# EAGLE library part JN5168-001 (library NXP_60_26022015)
JenNet, ZigBee PRO and IEEE802.15.4 Module The JN5168-001-Myy family is a range of ultra low power, high performance surface mount modules targeted at IEEE 802.15.4, JenNet-IP, ZigBee Light Link, ZigBee Smart Energy and RF4CE networking applications, enabling users to realise products with minimum time to market and at the lowest cost. They remove the need for expensive and lengthy development of custom RF board designs and test suites. The modules use NXP’s JN5168 wireless microcontroller to provide a comprehensive solution with large memory, high CPU and radio performance and all RF components included. All that is required to develop and manufacture wireless control or sensing products is to connect a power supply and peripherals such as switches, actuators and sensors, considerably simplifying product development. Four module variants are available: JN5168-001-M00 with an integrated antenna, JN5168-001- M03 with an antenna connector and the JN5168-001-M05 and M06 with an antenna connector, power amplifier and LNA for extended range. The JN5168-001-M05 output power has been optimised for use in Europe and Asia. AAL Eindhoven MK
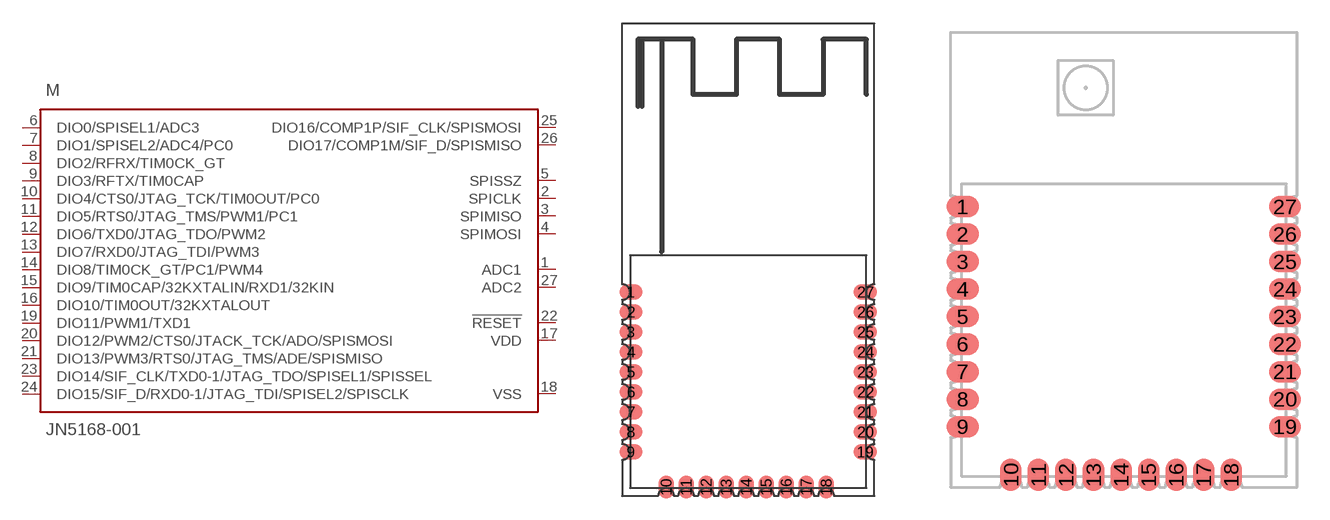
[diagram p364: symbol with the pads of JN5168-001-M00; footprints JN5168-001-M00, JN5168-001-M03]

Designator prefix M

## JN5168-001-M00 (DIO2: OK; DIO3: OK)  [JN5168-001-M00]
1  ADC1  pas
2  SPICLK  out
3  SPIMISO  in
4  SPIMOSI  in
5  SPISSZ  out
6  DIO0/SPISEL1/ADC3
7  DIO1/SPISEL2/ADC4/PC0
8  DIO2/RFRX/TIM0CK_GT
9  DIO3/RFTX/TIM0CAP
10  DIO4/CTS0/JTAG_TCK/TIM0OUT/PC0
11  DIO5/RTS0/JTAG_TMS/PWM1/PC1
12  DIO6/TXD0/JTAG_TDO/PWM2
13  DIO7/RXD0/JTAG_TDI/PWM3
14  DIO8/TIM0CK_GT/PC1/PWM4
15  DIO9/TIM0CAP/32KXTALIN/RXD1/32KIN
16  DIO10/TIM0OUT/32KXTALOUT
17  VDD
18  VSS  pwr
19  DIO11/PWM1/TXD1
20  DIO12/PWM2/CTS0/JTACK_TCK/ADO/SPISMOSI
21  DIO13/PWM3/RTS0/JTAG_TMS/ADE/SPISMISO
22  !RESET!  in
23  DIO14/SIF_CLK/TXD0-1/JTAG_TDO/SPISEL1/SPISSEL
24  DIO15/SIF_D/RXD0-1/JTAG_TDI/SPISEL2/SPISCLK
25  DIO16/COMP1P/SIF_CLK/SPISMOSI
26  DIO17/COMP1M/SIF_D/SPISMISO
27  ADC2  pas

## JN5168-001-M03 (DIO2: OK; DIO3: OK)  [JN5168-001-M03]
Pads as for JN5168-001-M00

## JN5168-001-M06 (DIO2: x; DIO3: x)  [JN5168-001-M06]
Pads as for JN5168-001-M00

## JN5168-001-M05 (DIO2: x; DIO3: x)  [JN5168-001-M06]
Pads as for JN5168-001-M00

## Footprint JN5168-001-M00 (pad centres in mm)
smd 1.5 x 1: 1 -7.44,2.45; 2 -7.44,1.18; 3 -7.44,-0.09; 4 -7.44,-1.36; 5 -7.44,-2.63; 6 -7.44,-3.9; 7 -7.44,-5.17; 8 -7.44,-6.44; 9 -7.44,-7.71; 19 7.44,-7.71; 20 7.44,-6.44; 21 7.44,-5.17; 22 7.44,-3.9; 23 7.44,-2.63; 24 7.44,-1.36; 25 7.44,-0.09; 26 7.44,1.18; 27 7.44,2.45
smd 1 x 1.5: 10 -5.21,-9.94; 11 -3.94,-9.94; 12 -2.67,-9.94; 13 -1.4,-9.94; 14 -0.13,-9.94; 15 1.14,-9.94; 16 2.41,-9.94; 17 3.68,-9.94; 18 4.95,-9.94

## Footprint JN5168-001-M03 (pad centres in mm)
JN5168-001-M03 %Descr% JEDEC: -- IEC: -- JEITA: --
smd 1.5 x 1: 1 -7.44,2.45; 2 -7.44,1.18; 3 -7.44,-0.09; 4 -7.44,-1.36; 5 -7.44,-2.63; 6 -7.44,-3.9; 7 -7.44,-5.17; 8 -7.44,-6.44; 9 -7.44,-7.71; 19 7.44,-7.71; 20 7.44,-6.44; 21 7.44,-5.17; 22 7.44,-3.9; 23 7.44,-2.63; 24 7.44,-1.36; 25 7.44,-0.09; 26 7.44,1.18; 27 7.44,2.45
smd 1 x 1.5: 10 -5.21,-9.94; 11 -3.94,-9.94; 12 -2.67,-9.94; 13 -1.4,-9.94; 14 -0.13,-9.94; 15 1.14,-9.94; 16 2.41,-9.94; 17 3.68,-9.94; 18 4.95,-9.94

## Footprint JN5168-001-M06 (pad centres in mm)
smd 1.5 x 1: 1 -7.44,2.45; 2 -7.44,1.18; 3 -7.44,-0.09; 4 -7.44,-1.36; 5 -7.44,-2.63; 6 -7.44,-3.9; 7 -7.44,-5.17; 8 -7.44,-6.44; 9 -7.44,-7.71; 19 7.44,-7.71; 20 7.44,-6.44; 21 7.44,-5.17; 22 7.44,-3.9; 23 7.44,-2.63; 24 7.44,-1.36; 25 7.44,-0.09; 26 7.44,1.18; 27 7.44,2.45
smd 1 x 1.5: 10 -5.21,-9.94; 11 -3.94,-9.94; 12 -2.67,-9.94; 13 -1.4,-9.94; 14 -0.13,-9.94; 15 1.14,-9.94; 16 2.41,-9.94; 17 3.68,-9.94; 18 4.95,-9.94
